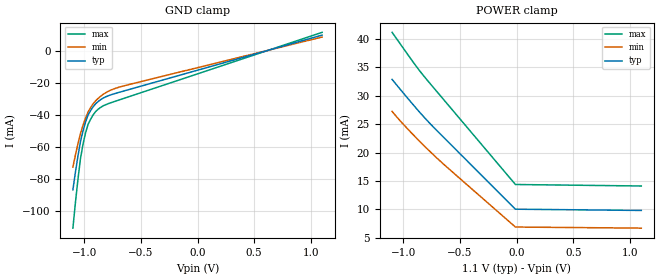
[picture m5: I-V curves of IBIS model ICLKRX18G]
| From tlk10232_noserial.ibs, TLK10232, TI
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[Model]   ICLKRX18G
Model_type   Input
Polarity   Non-Inverting
Vinl =  0.55
Vinh =  0.98
C_comp   0.222256p   0.1242037p   0.3440809p
[Model Spec]
Vinl   0.55   0.495   0.605
Vinh   0.98   0.98   0.98
[Temperature Range]   25   125   -40
[Voltage Range]   1.1   0.99   1.21
[POWER_clamp]
-1.1V     32.88mA    27.24mA    41.16mA
-1V       30.46mA    24.95mA    38.33mA
-866.7mV  27.32mA    22.18mA    34.65mA
-733.3mV  24.45mA    19.56mA    31.41mA
-11.11mV  10.02mA    6.877mA    14.37mA
1.1V      9.798mA    6.683mA    14.11mA
[GND_clamp]
-1.1V     -86.96mA   -72.73mA   -110.9mA
-1.078V   -75.93mA   -65.18mA   -94.94mA
-1.056V   -65.88mA   -58.19mA   -80.47mA
-1.033V   -56.81mA   -51.76mA   -67.51mA
-1.011V   -50.14mA   -46.63mA   -58.58mA
-988.9mV  -44.62mA   -42.16mA   -51.45mA
-966.7mV  -40.24mA   -38.34mA   -46.14mA
-922.2mV  -35.1mA    -33.28mA   -40.21mA
-877.8mV  -31.79mA   -29.81mA   -36.61mA
-788.9mV  -28.17mA   -25.41mA   -33.12mA
-677.8mV  -25.7mA    -22.48mA   -30.43mA
1.1V      9.798mA    8.6mA      11.51mA
